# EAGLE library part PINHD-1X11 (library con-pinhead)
PIN HEADER
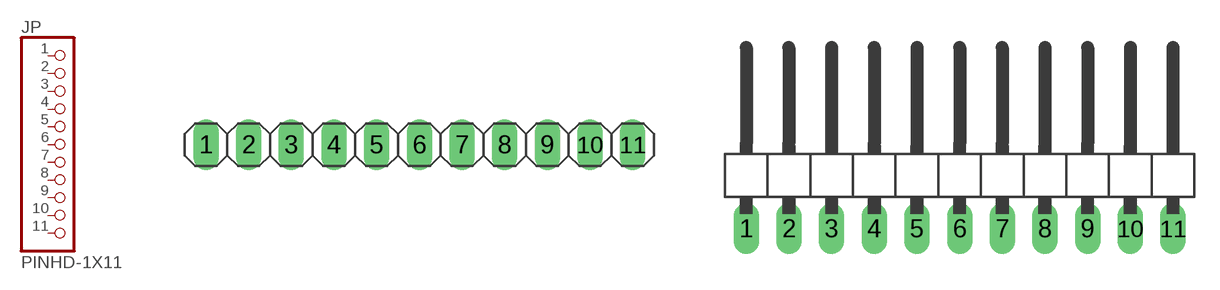
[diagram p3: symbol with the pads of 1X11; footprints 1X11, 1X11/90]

Designator prefix JP

## PINHD-1X11_2.54  [1X11]
1  1  pas
2  2  pas
3  3  pas
4  4  pas
5  5  pas
6  6  pas
7  7  pas
8  8  pas
9  9  pas
10  10  pas
11  11  pas

## PINHD-1X11_2.54-90°  [1X11/90]
Pads as for 1X11

## PINHD-1X11_2.00  [1X11M]
Pads as for 1X11

## PINHD-1X11_2.54-SMD  [1X11SMD]
Pads as for 1X11

## PINHD-1X11_2.54-SMD-90°  [1X11SMD/90]
Pads as for 1X11

## Footprint 1X11 (pad centres in mm)
PIN HEADER - 2.54
drill 1.016 long: 1 -12.7,0; 2 -10.16,0; 3 -7.62,0; 4 -5.08,0; 5 -2.54,0; 6 0,0; 7 2.54,0; 8 5.08,0; 9 7.62,0; 10 10.16,0; 11 12.7,0

## Footprint 1X11/90 (pad centres in mm)
PIN HEADER - 2.54 90°
drill 1.016 long: 1 -12.7,-3.81; 2 -10.16,-3.81; 3 -7.62,-3.81; 4 -5.08,-3.81; 5 -2.54,-3.81; 6 0,-3.81; 7 2.54,-3.81; 8 5.08,-3.81; 9 7.62,-3.81; 10 10.16,-3.81; 11 12.7,-3.81

## Footprint 1X11M (pad centres in mm)
PIN HEADER - 2
drill 0.914 square: 1 -10,0
drill 0.914: 2 -8,0; 3 -6,0; 4 -4,0; 5 -2,0; 6 0,0; 7 2,0; 8 4,0; 9 6,0; 10 8,0; 11 10,0

## Footprint 1X11SMD (pad centres in mm)
PIN HEADER - 2.54 SMD
smd 1.016 x 3.302: 1 -1.27,1.27; 2 1.27,-1.27; 3 3.81,1.27; 4 6.35,-1.27; 5 8.89,1.27; 6 11.43,-1.27; 7 13.97,1.27; 8 16.51,-1.27; 9 19.05,1.27; 10 21.59,-1.27; 11 24.13,1.27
